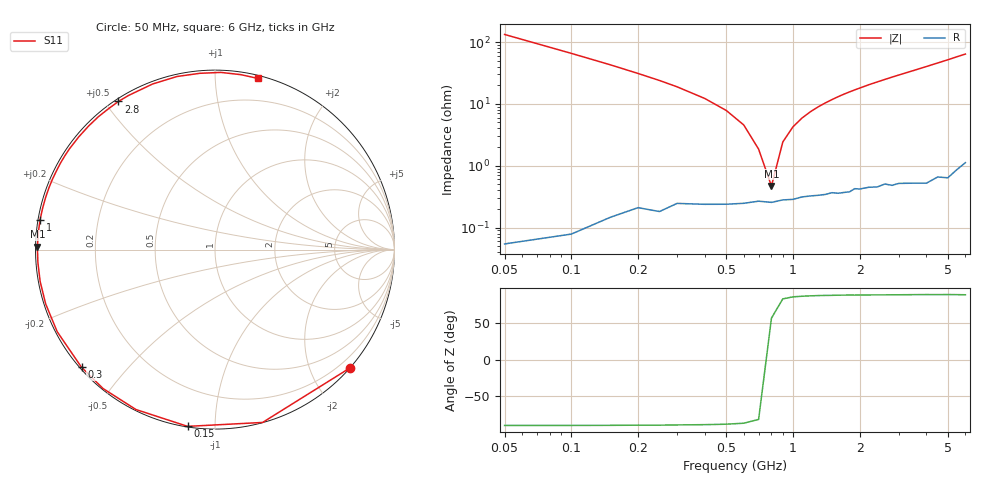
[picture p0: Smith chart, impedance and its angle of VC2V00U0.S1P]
! Infineon Technologies  Discrete & RF Semiconductors
! BBY 56-03
! Si Tuning Diode in SOD323
! VR = 2 V
! S-Parameters:  June  1999
# GHz  S  MA  R  50
!  f  S11
! GHz  MAG  ANG
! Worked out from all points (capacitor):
!   34 points, 50 MHz to 6 GHz, reference 50 ohm
!   read as one part to ground: C = 23.9 pF near 50 MHz
!   lowest |Z| = 468 mohm at 800 MHz (marker M1)
!   series resonance near 782.4 MHz, so ESL is about 1.7 nH
!   S11 on the Smith chart (normalised r, x): 50 MHz: 0.00, -2.65; 150 MHz: 0.00, -0.86; 300 MHz: 0.00, -0.38; 1 GHz: 0.01, +0.08; 2.8 GHz: 0.01, +0.54; 6 GHz: 0.02, +1.28
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0.05  0.9997 -41.3
0.1  0.9989 -74.6
0.15  0.9966 -98.8
0.2  0.994 -116.3
0.25  0.9941 -128.9
0.3  0.9914 -138.6
0.4  0.9911 -152.5
0.5  0.9908 -162.2
0.6  0.9903 -169.6
0.7  0.9894 -175.8
0.8  0.9899 179.1
0.9  0.9889 174.5
1  0.9887 170.3
1.1  0.9878 166.5
1.3  0.9872 159.7
1.6  0.9867 150.7
1.8  0.9863 145.3
2  0.9852 140.4
2.2  0.9848 135.6
2.4  0.985 131.3
2.8  0.9852 123.1
3  0.9847 119.3
3.5  0.986 110.6
4  0.9874 102.4
4.5  0.9858 94.9
5  0.9878 88.1
5.5  0.9853 81.6
6  0.9832 76.0
